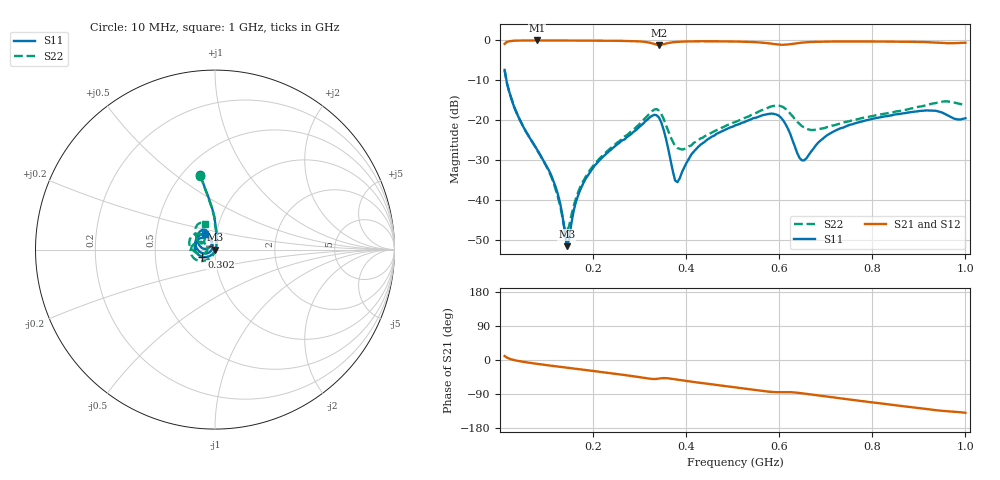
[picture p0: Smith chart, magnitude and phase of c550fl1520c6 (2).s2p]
!Agilent Technologies,N5234A,MY52241123,A.10.00.00
!Agilent N5234A: A.10.00.00
!Date: Wednesday, November 28, 2018 09:49:58
!Correction: S11(Full 2 Port(1,2))
!S21(Full 2 Port(1,2))
!S12(Full 2 Port(1,2))
!S22(Full 2 Port(1,2))
!S2P File: Measurements: S11, S21, S12, S22:
# Hz S  dB  R 50
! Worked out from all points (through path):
!   201 points, 10 MHz to 1 GHz, reference 50 ohm
!   highest |S21| = -0.07 dB at 79.3 MHz (marker M1); lowest = -1.2 dB at 341.6 MHz (marker M2)
!   group delay of S21, straight-line fit = 391 ps
!   lowest |S11| = -51.7 dB at 143.7 MHz (marker M3), VSWR 1.01, Z = 50.3 - j0.044 ohm
!   |S11| at or under -10 dB: 13.82 MHz to end of sweep
!   |S22| runs from -47.9 to -7.5 dB; largest |S21 - S12| = 0.0045
!   S11 on the Smith chart (normalised r, x): 10 MHz: 0.61, +0.62; 302.1 MHz: 0.86, -0.07; 1 GHz: 0.88, +0.16
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1e7  -7.46 101.3  -0.93 10.4  -0.93 10.5  -7.53 101.3
2.98e7  -16.54 89.6  -0.14 0.0  -0.14 -0.1  -16.53 90.2
7.93e7  -27.37 77.6  -0.07 -10.1  -0.08 -10.1  -27.51 78.1
1.2385e8  -38.40 57.9  -0.09 -17.2  -0.09 -17.2  -39.12 55.0
1.4365e8  -51.67 -9.7  -0.09 -20.3  -0.09 -20.3  -47.88 -23.8
1.6345e8  -40.44 -100.2  -0.10 -23.4  -0.10 -23.4  -39.58 -89.2
1.783e8  -36.07 -109.5  -0.11 -25.6  -0.11 -25.6  -35.46 -99.3
2.179e8  -29.63 -121.7  -0.13 -31.7  -0.13 -31.7  -29.23 -111.5
3.0205e8  -21.48 -152.8  -0.33 -45.7  -0.33 -45.7  -20.77 -136.0
3.4165e8  -19.40 145.1  -1.18 -49.0  -1.18 -49.0  -17.68 172.1
3.763e8  -35.21 144.9  -0.46 -50.9  -0.47 -50.9  -26.52 158.3
3.8125e8  -35.61 166.4  -0.42 -51.8  -0.42 -51.8  -27.06 165.1
4.258e8  -26.77 -154.0  -0.28 -59.5  -0.29 -59.5  -25.17 -162.7
5.05e8  -21.40 -171.2  -0.34 -72.2  -0.35 -72.2  -20.54 -166.3
5.941e8  -18.66 137.4  -1.04 -84.9  -1.04 -84.9  -16.36 157.5
6.139e8  -21.12 115.1  -1.12 -84.8  -1.13 -84.8  -17.25 140.1
6.4855e8  -30.12 136.5  -0.62 -87.8  -0.63 -87.8  -21.54 134.0
6.733e8  -27.25 172.2  -0.44 -91.9  -0.44 -91.9  -22.53 145.7
7.228e8  -22.55 172.3  -0.33 -100.0  -0.33 -100.0  -21.18 155.7
8.3665e8  -18.93 149.9  -0.35 -117.4  -0.36 -117.4  -18.23 147.4
9.307e8  -17.67 124.2  -0.57 -131.6  -0.57 -131.6  -15.86 132.5
1e9  -19.58 122.7  -0.63 -139.2  -0.63 -139.2  -16.23 112.0
